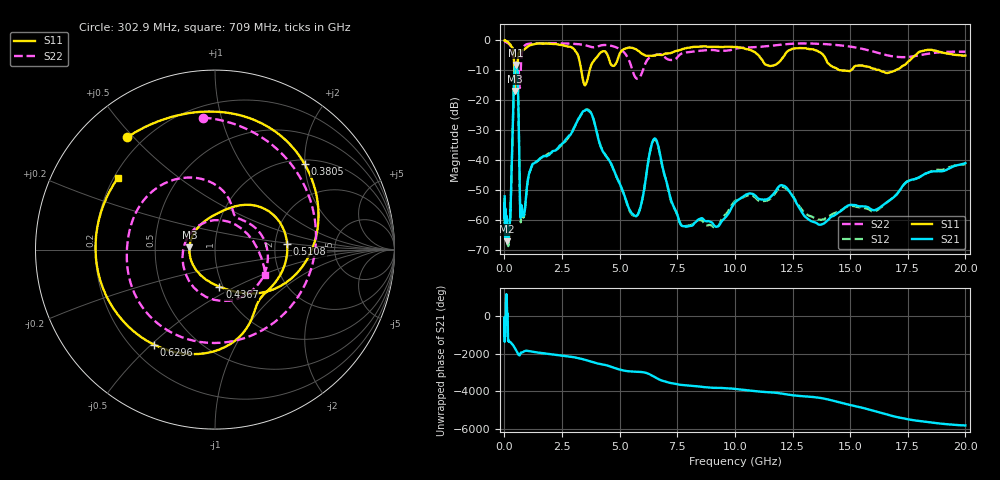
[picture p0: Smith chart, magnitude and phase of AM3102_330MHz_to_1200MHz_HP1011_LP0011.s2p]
! Date/Time: Tue, Sep 11, 2018 5:20 PM
! Network Analyzer: Agilent Technologies E8362B Rev: A.07.50.63
! Sweep from 0.010 to 20.000 GHz, 1601 Points, Sweep Type: LOG
! Power Supply: 4.949 V, 0.001 A
# Hz S DB R 50
!freq MagS11 AngS11 MagS21 AngS21 MagS12 AngS12 MagS22 AngS22
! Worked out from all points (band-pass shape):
!   1601 points, 10 MHz to 20 GHz, reference 50 ohm
!   highest |S21| = -8.21 dB at 491.8 MHz (marker M1); lowest = -67.0 dB at 125.2 MHz (marker M2)
!   |S21| within 3 dB of the highest: 430.1 MHz to 569.8 MHz (139.7 MHz wide, 27.9 % of centre)
!   lowest |S11| = -16.9 dB at 453.6 MHz (marker M3), VSWR 1.33, Z = 37.5 + j0.928 ohm
!   |S11| at or under -10 dB: 3.338 GHz to 3.695 GHz (356.3 MHz wide, 10.1 % of centre); 14.65 GHz to 15.02 GHz (373.4 MHz wide, 2.52 % of centre); 16.29 GHz to 16.95 GHz (659.2 MHz wide, 3.97 % of centre)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
!   |S22| runs from -15.8 to -0.1 dB; largest |S21 - S12| = 0.0044
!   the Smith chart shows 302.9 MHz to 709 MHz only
!   S11 on the Smith chart (normalised r, x): 302.9 MHz: 0.14, +0.48; 380.5 MHz: 1.10, +2.00; 436.7 MHz: 0.96, -0.42; 510.8 MHz: 2.34, +0.17; 629.6 MHz: 0.29, -0.51; 709 MHz: 0.22, +0.31
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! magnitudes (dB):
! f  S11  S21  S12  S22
! 10 MHz  0.0  -52.0  -53.2  -0.1
! 35.55 MHz  0.0  -62.0  -63.8  -0.3
! 125.2 MHz  -0.4  -67.0  -63.5  -0.8
! 126.4 MHz  -0.4  -66.0  -64.1  -0.8
! 197.5 MHz  -0.9  -63.2  -65.3  -1.1
! 302.9 MHz  -2.0  -46.4  -47.0  -2.6
! 380.5 MHz  -3.2  -22.3  -22.4  -5.6
! 436.7 MHz  -13.6  -10.3  -10.4  -6.0
! 447.2 MHz  -16.5  -9.3  -9.4  -6.1
! 453.6 MHz  -16.9  -8.9  -8.9  -6.2
! 491.8 MHz  -8.6  -8.2  -8.3  -6.5
! 510.8 MHz  -7.9  -8.2  -8.2  -7.5
! 629.6 MHz  -4.0  -30.7  -30.6  -10.8
! 709 MHz  -3.4  -59.2  -60.7  -10.1
! 1.59 GHz  -1.0  -39.1  -39.1  -0.9
! 3.634 GHz  -12.1  -23.3  -23.1  -1.9
! 5.652 GHz  -2.7  -58.5  -58.7  -11.9
! 6.518 GHz  -5.1  -32.7  -32.9  -4.9
! 7.92 GHz  -2.5  -62.1  -61.9  -4.0
! 12.03 GHz  -6.2  -48.3  -48.8  -1.4
! 13.81 GHz  -4.6  -61.3  -59.7  -1.2
! 20 GHz  -5.0  -40.9  -41.3  -3.7
